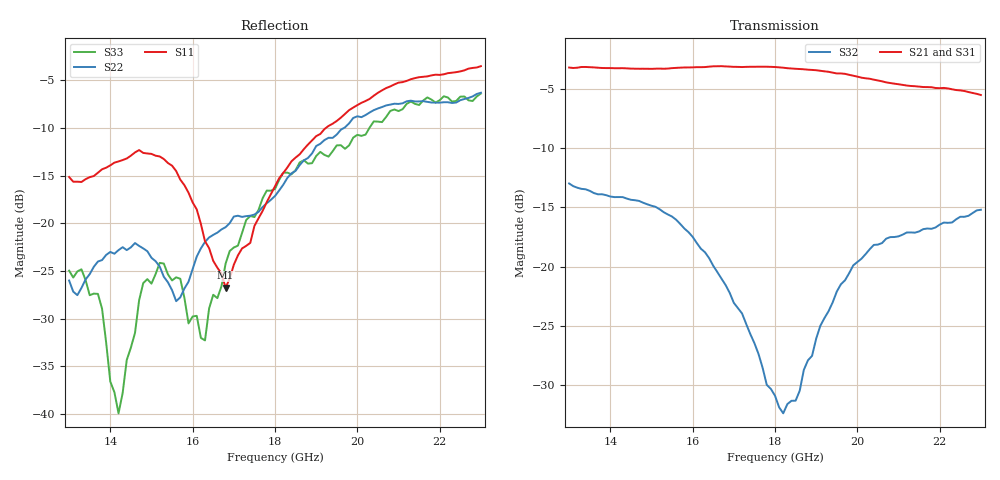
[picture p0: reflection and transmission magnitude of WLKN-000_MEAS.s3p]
! 7/15/2025 3:27:06 PM
! C:\MESURES\042-MESURES WLKN000 RO3006 STACK 1MM\DUT2528A2-WLKN000-8NU5P2.S3P
! CHANNEL.1
! TR.MEASUREMENT
! CORRECTED.DATA
! RF.CORRECTION: FULL.THREE.PORT.CAL.PORT.1.3.4
! AVERAGING.OFF
! IF.BANDWIDTH: 100HZ
! SWEEPTYPE:  FREQ.SWEEP(Linear)
! Reference Plane Port Info
! PORT:  PORT1  PORT3  PORT4
! DISTANCE:  0  m  0  m  0  m
! TIME:  0  s  0  s  0  s
! PHASE.OFFSET:  0  deg.  0  deg.  0  deg.
! LOSS:  0  dB  0  dB  0  dB
! REF.LOSS:  0  dB  0  dB  0  dB
! REF.FREQ:  0  Hz  0  Hz  0  Hz
! Power Info
! POWER:  -20  dBm  -20  dBm  -20  dBm
! EFF.POWER:  -20  dBm  -20  dBm  -20  dBm
! SOURCE.ATTEN:  0  dB  0  dB  0  dB
! TEST.ATTEN:  0  dB  0  dB  0  dB
# GHZ S RI R 50.0
! FREQ.GHZ  S11RE  S11IM  S13RE  S13IM  S14RE  S14IM
!  S31RE  S31IM  S33RE  S33IM  S34RE  S34IM
!  S41RE  S41IM  S43RE  S43IM  S44RE  S44IM
!; PortSelection: Port_134
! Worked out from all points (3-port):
!   101 points, 13 GHz to 23 GHz, reference 50 ohm
!   strongest paths, dB at 13 GHz, 15.5 GHz, 18 GHz, 20.5 GHz, 23 GHz:
!     S21: -3.2, -3.2, -3.1, -4.3, -5.5
!     S31: -3.2, -3.3, -3.2, -4.3, -5.6
!     S32: -13.0, -15.8, -30.9, -18.1, -15.2
!   lowest |S11| = -26.8 dB at 16.8 GHz (marker M1), VSWR 1.10, Z = 45.7 - j0.653 ohm
!   |S11| at or under -10 dB: start of sweep to 19.24 GHz
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13  0.1446 -0.0981  -0.3108 0.62  -0.2157 0.6521
    -0.3087 0.6199  0.0193 -0.0462  0.0396 0.2208
    -0.2179 0.6537  0.0396 0.2211  -0.0442 -0.0351
13.7  0.1295 -0.1307  -0.148 0.6756  -0.0388 0.6826
      -0.1467 0.6756  0.0595 -0.0207  0.085 0.1839
      -0.0379 0.6821  0.0844 0.1836  -0.0397 -0.0156
14.2  0.1234 -0.1709  -0.0189 0.6882  0.0862 0.6769
      -0.0192 0.6876  0.0698 0.0188  0.1162 0.1588
      0.0862 0.6757  0.1165 0.1586  -0.0086 0.00528
14.8  0.0966 -0.2128  0.1237 0.6726  0.2233 0.6423
      0.1243 0.673  0.0628 0.0388  0.1458 0.116
      0.2225 0.6416  0.1456 0.116  0.0455 0.017
15.6  0.0199 -0.1866  0.3109 0.617  0.4003 0.5592
      0.3111 0.6161  -0.00419 0.0388  0.1498 0.0484
      0.3993 0.5607  0.1501 0.0487  0.0492 0.0169
16.3  -0.0326 -0.0736  0.4651 0.5185  0.5423 0.4409
      0.4637 0.5186  -0.0678 0.0421  0.115 0.00488
      0.5426 0.4419  0.115 0.00462  0.00791 0.023
16.8  -0.0453 -0.00714  0.5575 0.4233  0.6182 0.3266
      0.5583 0.4225  -0.0731 0.0612  0.0835 -0.00638
      0.6182 0.3264  0.0835 -0.0061  -0.0128 0.06
18  -0.0585 0.1449  0.6857 0.1188  0.6897 0.00282
    0.6857 0.1193  0.00151 0.1389  0.0279 0.00573
    0.6896 0.00164  0.028 0.0058  0.0394 0.1459
20.8  0.4975 0.1557  0.3544 -0.4775  0.2398 -0.544
      0.3554 -0.478  0.2754 0.3153  0.0818 0.1056
      0.2398 -0.5444  0.0817 0.1054  0.362 0.1392
23  0.5814 -0.3241  -0.0925 -0.5212  -0.1866 -0.4888
    -0.0936 -0.522  0.4758 -0.083  0.1737 -0.012
    -0.1881 -0.489  0.1735 -0.0121  0.4669 -0.1053
